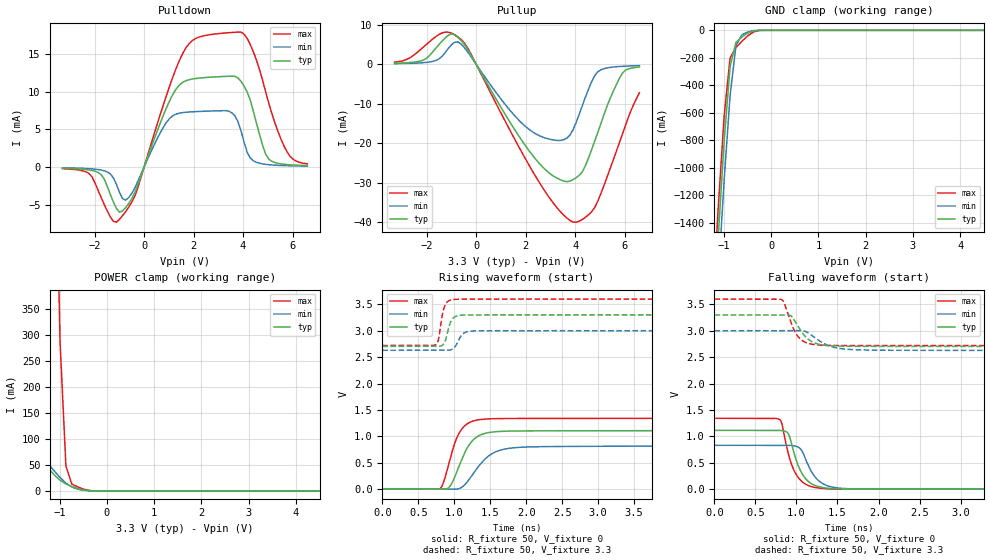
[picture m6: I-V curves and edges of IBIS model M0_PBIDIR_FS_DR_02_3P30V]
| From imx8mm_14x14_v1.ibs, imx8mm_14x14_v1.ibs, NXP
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|[Package Model]   There is an optional, fairly complex Package Modeling
|   section here in the file if you want it.  You will have
|   to add it yourself, because SiliconSmart has no
|   notion of packaging.  Please see the IBIS Specification
|   for details.
[Model] M0_PBIDIR_FS_DR_02_3P30V
Model_type I/O
Vinl  =  0.54
Vinh  =  1.26
Vmeas =  0.9
| Capacitance   typ   min   max
C_comp   2.08161232969e-12   2.03493647009e-12   2.16777276051e-12
| Variables   typ   min   max
[GND Clamp Reference]   0   0   0
[POWER Clamp Reference]   3.3   3   3.6
[Pulldown Reference]   0   0   0
[Pullup Reference]   3.3   3   3.6
[Temperature Range]   25   125   -40
[Voltage Range]   3.3   3   3.6
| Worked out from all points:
|   slope of the pulldown table from 0 to 0.495 V, typ, clamps not added: 111 ohm
|   slope of the pullup table from 0 to 0.495 V, typ, clamps not added: 90.9 ohm
|   GND clamp passes 1 mA (typ) near -0.28 V on its own axis
|   POWER clamp passes 1 mA (typ) near -0.44 V on its own axis
|   falling waveform, R_fixture 50, V_fixture 0: 20-80 % time 163ps typ, 180ps min, 156ps max; typ from 1.11 V to 0 V
|   falling waveform, R_fixture 50, V_fixture 3.3: 20-80 % time 175ps typ, 242ps min, 143ps max; typ from 3.3 V to 2.7 V
|   rising waveform, R_fixture 50, V_fixture 0: 20-80 % time 230ps typ, 318ps min, 191ps max; typ from 0 V to 1.11 V
|   rising waveform, R_fixture 50, V_fixture 3.3: 20-80 % time 76.1ps typ, 93.5ps min, 65.6ps max; typ from 2.7 V to 3.3 V
[GND Clamp]
| Voltage   I(typ)   I(min)   I(max)
-3.3V     -15.63A    -15.86A    -15.46A
-1.241V   -2.232A    -2.527A    -2.015A
-1.117V   -1.487A    -1.785A    -1.276A
-993.1mV  -798.9mA   -1.083A    -616.8mA
-869mV    -263.4mA   -475.6mA   -200.8mA
-744.8mV  -87.36mA   -112.1mA   -126.1mA
-620.7mV  -49.17mA   -33.01mA   -80.34mA
-496.6mV  -20.8mA    -11.81mA   -40.7mA
-372.4mV  -3.877mA   -2.002mA   -11.64mA
-248.3mV  -117.5uA   -105.1uA   -542.9uA
6.6V      0A         0A         0A
[POWER Clamp]
| Voltage   I(typ)   I(min)   I(max)
-3.3V     11.6A      9.427A     14.09A
-1.862V   2.37A      558.5mA    4.855A
-1.738V   1.676A     202.6mA    4.157A
-1.614V   1.03A      99.77mA    3.468A
-1.49V    451mA      80.49mA    2.786A
-1.366V   91.11mA    66.06mA    2.111A
-1.241V   43.77mA    52.06mA    1.45A
-1.117V   30.97mA    38.55mA    817.5mA
-993.1mV  20.41mA    25.92mA    286.6mA
-869mV    13.37mA    15.08mA    47.85mA
-744.8mV  8.524mA    7.507mA    13.32mA
6.6V      0A         0A         0A
[Pulldown]
| Voltage   I(typ)   I(min)   I(max)
-3.3V     -168.2uA   -115.7uA   -233.4uA
-2.234V   -392.9uA   -232.7uA   -861.2uA
-1.738V   -1.023mA   -416.8uA   -4.059mA
-1.117V   -5.529mA   -2.354mA   -7.34mA
-620.7mV  -4.853mA   -4.065mA   -5.331mA
910.3mV   7.901mA    5.941mA    9.566mA
1.707V    11.46mA    7.262mA    15.89mA
3.797V    11.81mA    6.011mA    17.9mA
4.293V    8.862mA    1.179mA    16.25mA
5.038V    1.051mA    295.3uA    8.479mA
5.783V    309uA      164uA      1.983mA
6.6V      174uA      109.6uA    405.1uA
[Pullup]
| Voltage   I(typ)   I(min)   I(max)
-3.3V     289.4uA    183.1uA    562.7uA
-2.11V    1.149mA    447.4uA    4.519mA
-1.366V   5.986mA    2.154mA    8.003mA
-993.1mV  7.726mA    5.014mA    7.907mA
-620.7mV  6.113mA    5.204mA    6.351mA
2.162V    -22.08mA   -16.58mA   -25.8mA
3.3V      -28.92mA   -19.28mA   -36.56mA
3.921V    -29.18mA   -16.51mA   -39.93mA
4.293V    -27.18mA   -10.43mA   -39.28mA
4.914V    -17.28mA   -1.899mA   -34.69mA
5.907V    -2.264mA   -494.8uA   -17.76mA
6.6V      -659.9uA   -331.9uA   -7.186mA
[Ramp]
dV/dt_r   0.668087/0.230367n  0.49733/0.318236n  0.805158/0.190549n
dV/dt_f   0.357579/0.174657n  0.222408/0.241737n  0.527482/0.142722n
R_load = 50
[Falling Waveform]
R_fixture = 50
V_fixture = 0
V_fixture_min = 0
V_fixture_max = 0
| Time   V(typ)   V(min)   V(max)
0s        1.114V     831.1mV    1.342V
791.1ps   1.113V     831.1mV    1.323V
824.1ps   1.109V     831.1mV    1.226V
903.9ps   1.042V     830.3mV    650.1mV
972.1ps   676.1mV    819.9mV    350.4mV
1.059ns   318.5mV    743.1mV    153.5mV
1.181ns   104.9mV    334.2mV    48.26mV
1.29ns    39.32mV    136mV      17.2mV
1.697ns   963.9uV    4.684mV    -206.8uV
333.3ns   4.253uV    5.92uV     19.88uV
[Falling Waveform]
R_fixture = 50
V_fixture = 3.3
V_fixture_min = 3
V_fixture_max = 3.6
| Time   V(typ)   V(min)   V(max)
0s        3.3V       3V         3.6V
813.4ps   3.301V     3V         3.595V
845.7ps   3.301V     3V         3.541V
936.9ps   3.279V     3.001V     3.138V
1ns       3.136V     3.001V     2.933V
1.073ns   2.959V     3.001V     2.812V
1.258ns   2.751V     2.833V     2.732V
1.424ns   2.715V     2.7V       2.723V
1.642ns   2.706V     2.647V     2.721V
333.3ns   2.704V     2.629V     2.721V
[Rising Waveform]
R_fixture = 50
V_fixture = 0
V_fixture_min = 0
V_fixture_max = 0
| Time   V(typ)   V(min)   V(max)
0s        4.252uV    5.918uV    19.88uV
800.2ps   -202.7uV   -17.31uV   9.787mV
855.9ps   -817.7uV   -18.93uV   151mV
947.9ps   69.7mV     -390uV     605.9mV
1.043ns   351.8mV    1.137mV    994mV
1.142ns   682.6mV    79.04mV    1.195V
1.285ns   959.3mV    335.7mV    1.299V
1.487ns   1.073V     637mV      1.331V
1.872ns   1.101V     788.2mV    1.338V
333.3ns   1.113V     828.9mV    1.342V
[Rising Waveform]
R_fixture = 50
V_fixture = 3.3
V_fixture_min = 3
V_fixture_max = 3.6
| Time   V(typ)   V(min)   V(max)
0s        2.704V     2.629V     2.721V
739.4ps   2.704V     2.629V     2.733V
777.5ps   2.704V     2.629V     2.819V
839.2ps   2.728V     2.629V     3.34V
889.6ps   2.876V     2.63V      3.525V
937ps     3.125V     2.635V     3.577V
982.3ps   3.235V     2.658V     3.592V
1.101ns   3.295V     2.916V     3.599V
1.182ns   3.299V     2.982V     3.6V
333.3ns   3.3V       3V         3.6V
